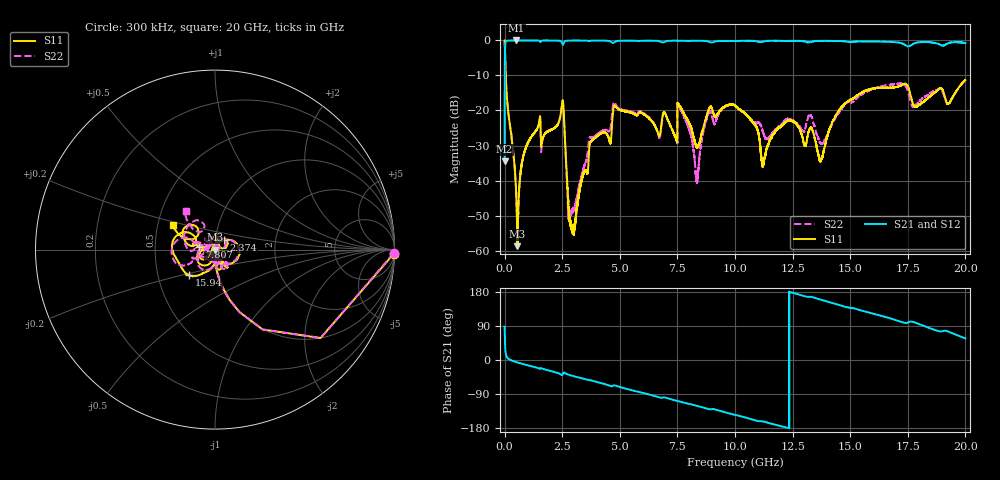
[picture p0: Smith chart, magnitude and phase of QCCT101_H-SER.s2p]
! Created Fri Feb  5 15:30:39 2021
# hz S ma R 50
! 2 Port Network Data from SP1.SP block
! freq  magS11  angS11  magS21  angS21  magS12  angS12  magS22  angS22
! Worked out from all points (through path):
!   20001 points, 300 kHz to 20 GHz, reference 50 ohm
!   highest |S21| = -0.01 dB at 510.3 MHz (marker M1); lowest = -34.5 dB at 300 kHz (marker M2)
!   group delay of S21, straight-line fit = 41.8 ps
!   lowest |S11| = -58.7 dB at 559.3 MHz (marker M3), VSWR 1.00, Z = 49.9 + j0.0163 ohm
!   |S11| at or under -10 dB: 47.56 MHz to end of sweep
!   |S22| runs from -58.1 to 0.0 dB; largest |S21 - S12| = 0.014
!   S11 on the Smith chart (normalised r, x): 300 kHz: 10, -90; 2.374 GHz: 1.10, +0.11; 7.807 GHz: 0.84, +0.02; 15.94 GHz: 0.72, -0.21; 20 GHz: 0.60, +0.18
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300000  0.9976 -1.3  0.01878 88.0  0.01881 88.6  0.9948 -1.2
1.083e8  0.142 -83.4  0.9887 6.8  0.9893 6.8  0.1429 -83.4
5.103e8  0.005826 -108.6  0.9994 -5.6  0.9973 -5.6  0.005616 -108.4
5.593e8  0.001156 171.9  0.999 -6.5  0.9984 -6.5  0.001375 171.1
1.0413e9  0.0362 77.2  0.9984 -14.5  0.9983 -14.5  0.0363 76.9
2.3743e9  0.07158 46.0  0.9876 -36.1  0.988 -36.1  0.07158 50.1
2.5493e9  0.1203 -40.3  0.8808 -34.0  0.8806 -34.0  0.1145 -42.9
2.7593e9  0.005439 -58.7  0.9934 -38.4  0.9938 -38.3  0.003441 -61.3
2.9103e9  0.002031 43.6  0.9963 -41.2  0.9964 -41.2  0.003489 0.9
3.3343e9  0.009715 -174.9  0.997 -48.1  0.9972 -48.0  0.0116 -92.5
4.7803e9  0.1171 -143.2  0.9519 -66.9  0.9532 -66.9  0.1286 -134.3
6.6673e9  0.04673 -165.1  0.9823 -97.8  0.982 -97.8  0.04577 -178.1
7.8073e9  0.08738 171.4  0.9868 -113.1  0.9875 -113.1  0.0786 153.2
8.3503e9  0.02945 -128.8  0.9891 -121.1  0.9908 -121.0  0.01036 51.5
8.8573e9  0.102 -67.8  0.9626 -129.7  0.9626 -129.6  0.09191 -51.2
1.00003e10  0.1181 -57.5  0.9787 -144.8  0.9799 -144.9  0.1183 -65.6
1.12183e10  0.01656 142.1  0.9654 -162.0  0.9645 -162.1  0.04883 173.1
1.33343e10  0.05522 92.3  0.9606 166.3  0.9595 166.2  0.07951 111.1
1.37343e10  0.01984 -11.7  0.9852 158.8  0.9858 158.9  0.03393 142.0
1.59433e10  0.2042 -135.7  0.9622 123.1  0.9642 123.1  0.1983 -153.5
1.66673e10  0.2104 -152.6  0.955 111.1  0.9471 110.9  0.2308 -161.1
2e10  0.2716 150.0  0.9144 57.1  0.9077 56.9  0.2716 127.2
